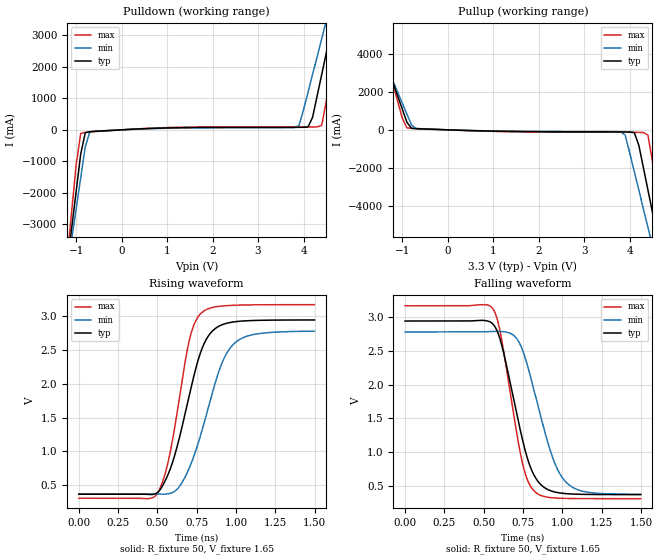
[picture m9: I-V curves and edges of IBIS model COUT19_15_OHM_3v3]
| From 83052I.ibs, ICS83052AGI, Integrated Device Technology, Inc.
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[Model] COUT19_15_OHM_3v3
Model_type   Output
Polarity   Non-Inverting
|   typ   min   max
C_comp   2pF   1.5pF   2.5pF
Vmeas = 1.65V
Rref = 50
Cref = 0
Vref = 1.65V
|   typ   min   max
[Voltage range]   3.3V   3.135V   3.465V
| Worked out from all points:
|   slope of the pulldown table from 0 to 0.495 V, typ, clamps not added: 13.8 ohm
|   slope of the pullup table from 0 to 0.495 V, typ, clamps not added: 12.8 ohm
|   rising waveform, R_fixture 50, V_fixture 1.65: 20-80 % time 167ps typ, 189ps min, 127ps max; typ from 0.368 V to 2.94 V
|   falling waveform, R_fixture 50, V_fixture 1.65: 20-80 % time 150ps typ, 172ps min, 123ps max; typ from 2.94 V to 0.368 V
[Pulldown]
|Voltage   I (typ)   I (min)   I (max)
-3.3V     -29.16A    -25.19A    -35.83A
-1.2V     -4.318A    -4.479A    -4.126A
-1.1V     -3.135A    -3.493A    -2.615A
-900mV    -768.5mA   -1.522A    -115.3mA
-800mV    -92.64mA   -536.7mA   -79.85mA
-700mV    -59.09mA   -73.31mA   -66.33mA
3.9V      79.76mA    136mA      91.46mA
4.2V      402.1mA    1.761A     92.61mA
4.4V      1.755A     2.891A     141.7mA
4.6V      3.111A     4.023A     1.761A
4.8V      4.47A      5.157A     3.494A
6.6V      16.85A     15.48A     19.28A
[Pullup]
|Voltage   I (typ)   I (min)   I (max)
-3.3V     16.79A     14.51A     20.63A
-1.7V     5.859A     5.382A     6.694A
-1.6V     5.176A     4.812A     5.823A
-900mV    397.4mA    826.4mA    100.6mA
-700mV    62.24mA    62.88mA    71.75mA
3.8V      -108.8mA   -105.6mA   -127.1mA
4.1V      -144.9mA   -2.201A    -130mA
4.3V      -1.996A    -4.167A    -145.4mA
4.4V      -3.176A    -5.151A    -274.3mA
4.6V      -5.537A    -7.119A    -3.192A
4.8V      -7.899A    -9.088A    -6.208A
6.6V      -29.16A    -26.82A    -33.35A
[Ramp]
|   typ   min   max
dV/dt_r   2.066/0.257n   1.929/0.292n   2.296/0.196n
dV/dt_f   2.07/0.226n   1.936/0.26n   2.304/0.182n
R_load =   50.0000
[Rising Waveform]
R_fixture = 50
V_fixture = 1.65   |Vcc_typ
V_fixture_min = 1.5675 |Vcc_min
V_fixture_max = 1.7325 |Vcc_max
C_fixture = 0.0p
| Time   typ   min   max
0s        367.7mV    370.7mV    307.4mV
498.5ps   389.3mV    370.2mV    373.4mV
567.6ps   660.5mV    373.5mV    844mV
642.6ps   1.232V     490.5mV    1.834V
711.7ps   1.924V     807.3mV    2.729V
785.3ps   2.533V     1.328V     3.061V
900.9ps   2.865V     2.253V     3.149V
992.5ps   2.919V     2.606V     3.163V
1.141ns   2.94V      2.742V     3.17V
1.498ns   2.945V     2.78V      3.172V
[Falling Waveform]
R_fixture = 50
V_fixture = 1.65   |Vcc_typ
V_fixture_min = 1.5675 |Vcc_min
V_fixture_max = 1.7325 |Vcc_max
C_fixture = 0.0p
| Time   typ   min   max
0s        2.945V     2.784V     3.172V
558.6ps   2.901V     2.792V     3.126V
608.1ps   2.642V     2.791V     2.747V
716.2ps   1.501V     2.664V     1.199V
768.8ps   980.2mV    2.362V     646.3mV
830.3ps   615.2mV    1.82V      401.2mV
941.4ps   413.2mV    898.7mV    319.8mV
1.032ns   380.9mV    534.7mV    311mV
1.165ns   370.5mV    402.4mV    308.2mV
1.498ns   367.8mV    372.3mV    307.5mV
